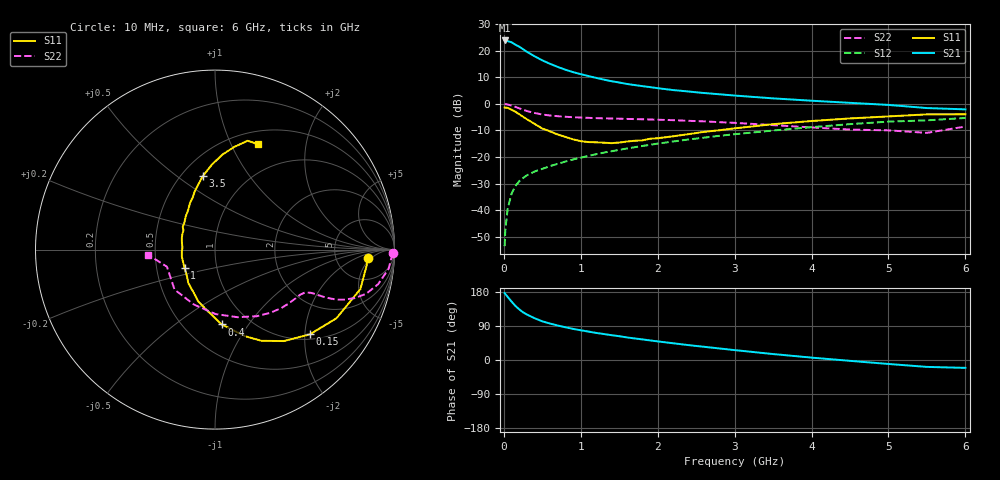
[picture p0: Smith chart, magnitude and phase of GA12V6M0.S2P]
! Infineon Technologies  Discrete & RF Semiconductors
! BF775
! Si NPN RF Bipolar Junction Transistor in SOT23
! VCE = 12 V  IC = 6 mA
! Common Emitter S-Parameters:  May  1996
# GHz  S  MA  R  50
!  f  S11  S21  S12  S22
! GHz  MAG  ANG  MAG  ANG  MAG  ANG  MAG  ANG
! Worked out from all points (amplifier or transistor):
!   36 points, 10 MHz to 6 GHz, reference 50 ohm
!   highest |S21| = 23.8 dB at 10 MHz (marker M1)
!   |S21| within 3 dB of that: start of sweep to 234.5 MHz
!   unconditionally stable (mu >= 1): 809.4 MHz to 2.842 GHz
!   at 250 MHz: K = 0.52, MSG = 24.2 dB, |S12| = -27.9 dB
!   at 1.4 GHz: K = 1.10, MAG = 11.2 dB, |S12| = -17.8 dB
!   at 6 GHz: K = 0.87, MSG = 1.6 dB, |S12| = -5.3 dB
!   S11 on the Smith chart (normalised r, x): 10 MHz: 11, -4; 150 MHz: 1.12, -2.12; 400 MHz: 0.75, -0.76; 1 GHz: 0.70, -0.15; 3.5 GHz: 0.63, +0.62; 6 GHz: 0.65, +1.28
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0.01  0.8522 -3.1  15.55 176.7  0.0021 79.7  0.9906 -1.2
0.02  0.8492 -6.1  15.13 173.9  0.0044 81.5  0.9843 -2.6
0.05  0.8393 -15.2  15.11 166.4  0.0106 82.3  0.9728 -6.4
0.1  0.7772 -29.5  14.36 154.2  0.0203 75.2  0.9287 -12.0
0.15  0.7085 -41.8  12.95 142.8  0.0285 68.6  0.8773 -16.3
0.2  0.6381 -53.0  11.87 133.7  0.035 65.6  0.8229 -19.2
0.25  0.5704 -63.0  10.64 125.8  0.0401 62.2  0.7709 -21.2
0.3  0.513 -70.5  9.492 119.9  0.0452 60.9  0.7317 -22.4
0.4  0.4187 -84.9  7.838 110.3  0.0533 59.9  0.6726 -23.4
0.5  0.3427 -97.2  6.562 102.1  0.0598 59.7  0.6291 -23.8
0.6  0.3031 -108.1  5.652 96.2  0.0673 60.3  0.6029 -24.0
0.7  0.2646 -117.3  4.947 91.0  0.0744 60.6  0.5849 -24.3
0.8  0.2388 -128.5  4.378 86.4  0.0819 60.8  0.5707 -24.8
1  0.1981 -148.8  3.61 78.4  0.097 61.8  0.5518 -25.9
1.1  0.1907 -159.0  3.324 75.0  0.1047 62.0  0.5444 -26.9
1.3  0.1855 -175.9  2.852 68.5  0.1207 61.9  0.5335 -28.7
1.6  0.1952 161.3  2.365 59.6  0.1446 61.1  0.52 -32.4
2.2  0.245 132.0  1.814 44.2  0.1953 58.2  0.4925 -41.5
3.5  0.4143 99.5  1.266 15.7  0.3143 46.8  0.3972 -71.5
4.5  0.531 85.5  1.043 -2.2  0.4147 35.3  0.3278 -111.1
5.5  0.6328 73.4  0.832 -18.2  0.4885 20.0  0.2843 -160.4
6  0.6351 67.7  0.786 -20.8  0.5418 15.9  0.3738 -175.6
